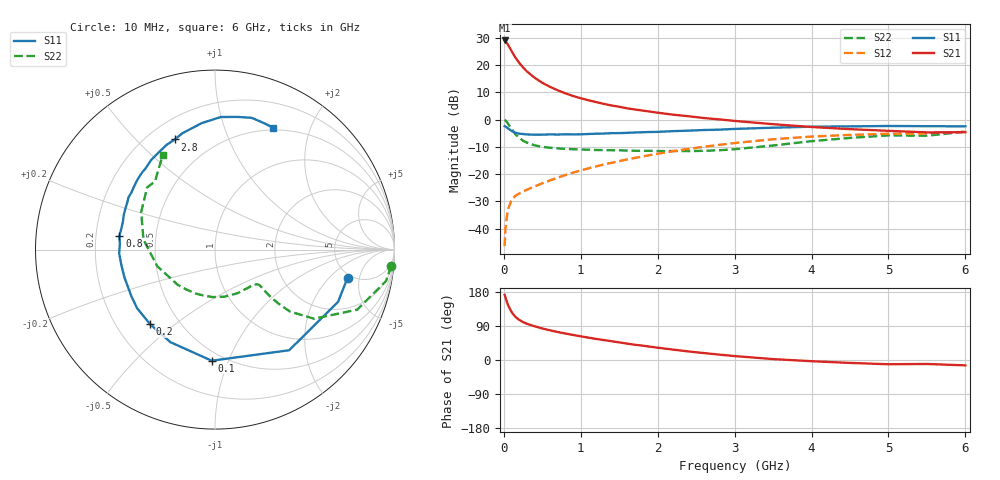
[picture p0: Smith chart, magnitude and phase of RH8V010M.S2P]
! SIEMENS Small Signal Semiconductors
! BFR106
! Si NPN RF Bipolar Junction Transistor in SOT23
! VCE = 8 V  IC = 10 mA
! Common Emitter S-Parameters:  August  1996
# GHz  S  MA  R  50
!  f  S11  S21  S12  S22
! GHz  MAG  ANG  MAG  ANG  MAG  ANG  MAG  ANG
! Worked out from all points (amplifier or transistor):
!   36 points, 10 MHz to 6 GHz, reference 50 ohm
!   highest |S21| = 29.0 dB at 10 MHz (marker M1)
!   |S21| within 3 dB of that: start of sweep to 82.9 MHz
!   unconditionally stable (mu >= 1): 489.2 MHz to 2.004 GHz; 5.378 GHz to end of sweep
!   at 250 MHz: K = 0.70, MSG = 22.7 dB, |S12| = -26.4 dB
!   at 1.4 GHz: K = 1.09, MAG = 8.7 dB, |S12| = -15.8 dB
!   at 6 GHz: K = 1.00, MAG = -0.5 dB, |S12| = -4.5 dB
!   S11 on the Smith chart (normalised r, x): 10 MHz: 4.65, -3.37; 100 MHz: 0.43, -0.87; 200 MHz: 0.34, -0.41; 800 MHz: 0.30, +0.06; 2.8 GHz: 0.31, +0.65; 6 GHz: 0.47, +1.48
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0.01  0.7553 -11.9  28.07 171.9  0.0048 85.3  0.9859 -5.3
0.02  0.745 -23.0  27.34 165.6  0.0098 79.1  0.9691 -10.4
0.05  0.6966 -53.6  23.87 147.0  0.0218 65.3  0.86 -22.9
0.1  0.6193 -91.7  18.06 126.8  0.0338 54.3  0.6728 -34.9
0.15  0.5724 -115.7  13.67 113.7  0.0401 48.3  0.5413 -39.6
0.2  0.5507 -131.1  10.94 106.0  0.0443 47.8  0.464 -40.4
0.25  0.5431 -143.0  8.974 99.8  0.0481 48.3  0.4087 -40.4
0.3  0.5335 -150.7  7.602 95.6  0.0518 50.0  0.3775 -40.1
0.4  0.5279 -162.6  5.836 89.0  0.0595 52.9  0.3372 -39.0
0.5  0.5288 -170.6  4.707 83.2  0.068 56.0  0.316 -38.6
0.6  0.5344 -177.9  3.971 78.3  0.0768 58.2  0.3043 -39.4
0.8  0.5379 172.0  3.018 69.9  0.0964 61.3  0.2894 -42.6
0.9  0.5347 167.7  2.7 66.1  0.1067 62.4  0.2862 -44.2
1.1  0.5437 159.2  2.256 59.0  0.1278 63.6  0.2803 -50.1
1.3  0.5539 152.2  1.935 52.6  0.1505 63.8  0.2754 -56.0
1.6  0.5708 142.4  1.607 43.3  0.1857 62.7  0.2703 -66.8
2.2  0.6131 125.4  1.228 27.4  0.263 57.9  0.265 -92.6
2.8  0.6533 110.1  1.007 14.2  0.344 50.0  0.274 -126.1
3.5  0.709 95.9  0.822 2.4  0.436 38.9  0.3348 -164.0
4.5  0.75 80.3  0.667 -7.7  0.5234 21.1  0.461 153.2
5.5  0.7553 68.3  0.582 -10.5  0.5583 8.9  0.5057 131.4
6  0.752 64.4  0.587 -14.2  0.5954 0.9  0.6004 119.1
